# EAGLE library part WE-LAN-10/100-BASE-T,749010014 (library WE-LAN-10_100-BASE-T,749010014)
LAN-Transformer WE-LAN 10/100 Base T - Compliant with IEEE 802.3 standards - SMD -- Ethernet -- Power over Ethernet -- 1 Gigabit Ethernet -- Compliant with most IC's for ethernet applications like Intel, AMD, Globespan and Realtek -- Hub, Router, Switch
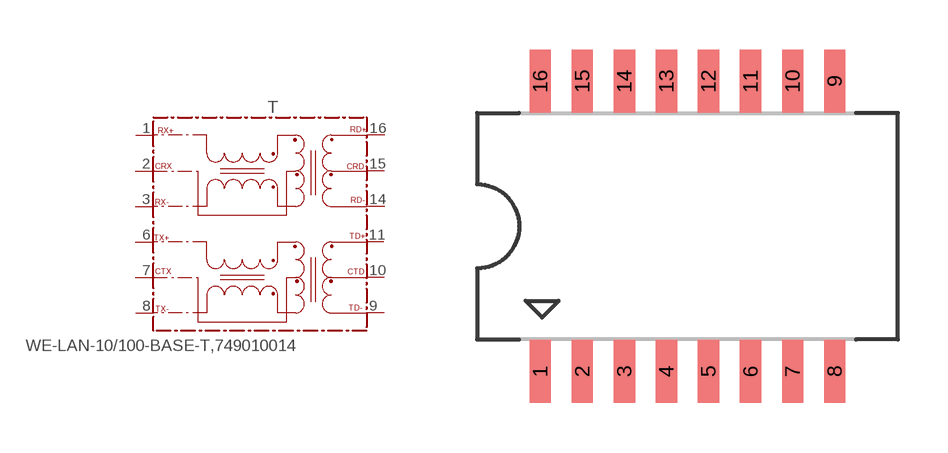
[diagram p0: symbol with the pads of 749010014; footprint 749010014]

Designator prefix T

## WE-LAN-10/100-BASE-T,749010014 (MPN: 749010014; OC_FARNELL: 1636347; OC_NEWARK: 08P2939; PACKAGE: 10/100/Base-T; SUPPLIER: Wuerth Elektronik)  [749010014]
1  RX+
2  CRX
3  RX-
6  TX+
7  CTX
8  TX-
9  TD-
10  CTD
11  TD+
14  RD-
15  CRD
16  RD+

## Footprint 749010014 (pad centres in mm)
MAX Height =5.08mm
smd 0.64 x 1.91: 1 -4.445,-4.385; 2 -3.175,-4.385; 3 -1.905,-4.385; 4 -0.635,-4.385; 5 0.635,-4.385; 6 1.905,-4.385; 7 3.175,-4.385; 8 4.445,-4.385; 9 4.445,4.385; 10 3.175,4.385; 11 1.905,4.385; 12 0.635,4.385; 13 -0.635,4.385; 14 -1.905,4.385; 15 -3.175,4.385; 16 -4.445,4.385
